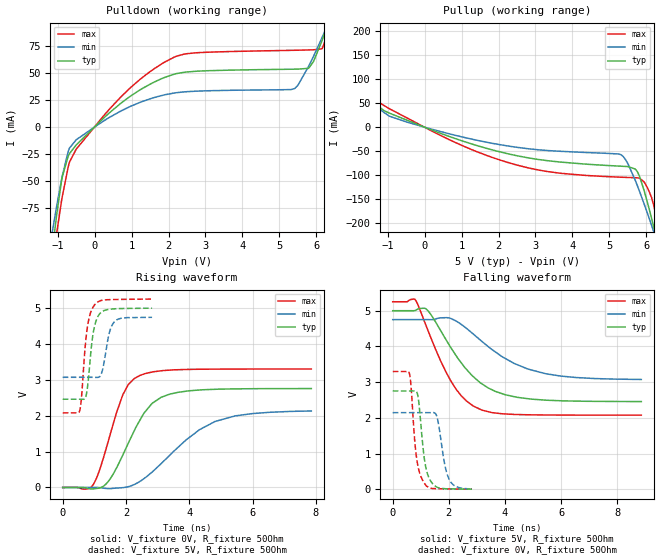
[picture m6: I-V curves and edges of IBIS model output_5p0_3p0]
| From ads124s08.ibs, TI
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|   output_5p0_3p0 Model
[Model]   output_5p0_3p0
Model_type   Output
Polarity   Non-Inverting
Vmeas = 2.5
Vref = 0
Cref = 2pF
Rref = 70
|   typ   min   max
|   (nom PVT)   (fast PVT)   (slow PVT)
C_comp   3.234e-12   3.122e-12   3.353e-12
| Where nom  PVT is Nominal Process, 5V, 27C
|   Fast PVT is Strong Process,  5.25V, -50C
|   Slow PVT is Weak Process,   4.75V, 125C
[Voltage Range]   5   4.75   5.25
|Junction Temperature
[Temperature Range]   27   125   -50
[Pullup Reference]   5   4.75   5.25
[Pulldown Reference]   0   0   0
[Power Clamp Reference]   5   4.75   5.25
[GND Clamp Reference]   0   0   0
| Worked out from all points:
|   slope of the pulldown table from 0 to 0.75 V, typ, clamps not added: 32.7 ohm
|   slope of the pullup table from 0 to 0.75 V, typ, clamps not added: 34.9 ohm
|   falling waveform, V_fixture 5V, R_fixture 50Ohm: 20-80 % time 1.48ns typ, 1.91ns min, 1.18ns max; typ from 5 V to 2.46 V
|   rising waveform, V_fixture 0V, R_fixture 50Ohm: 20-80 % time 988ps typ, 1.71ns min, 705ps max; typ from 0 V to 2.75 V
|   rising waveform, V_fixture 5V, R_fixture 50Ohm: 20-80 % time 199ps typ, 217ps min, 197ps max; typ from 2.46 V to 4.99 V
|   falling waveform, V_fixture 0V, R_fixture 50Ohm: 20-80 % time 237ps typ, 276ps min, 221ps max; typ from 2.75 V to 0.009 V
[Pulldown]
|   Voltage   I(typ)   I(min)   I(max)
-5V       -1.425A    -1.08A     -1.771A
-1.16V    -119.2mA   -100.1mA   -147mA
-1.015V   -78.19mA   -70.86mA   -95.57mA
-720mV    -27.41mA   -23.12mA   -37.56mA
-497mV    -16.44mA   -11.66mA   -20.31mA
905mV     27.09mA    18.18mA    34.43mA
2.225V    49.61mA    31.92mA    65.71mA
5.412V    53.62mA    35.7mA     71.12mA
5.79V     54.4mA     56.23mA    71.41mA
6.162V    80.92mA    83.39mA    72.89mA
6.403V    104.4mA    102.3mA    95.38mA
10V       508.4mA    415.8mA    608.3mA
[Pullup]
|   Voltage   I(typ)   I(min)   I(max)
-5V       423.9mA    339.6mA    534.5mA
-2.473V   163.8mA    135.3mA    202.2mA
-1.335V   51.05mA    46.44mA    59.22mA
-497mV    15.05mA    10.92mA    19.97mA
1.09V     -30.47mA   -21.72mA   -40.73mA
2.481V    -59.12mA   -41.74mA   -78.43mA
5.322V    -81.19mA   -57.63mA   -104mA
5.76V     -93.15mA   -122.3mA   -105.4mA
5.945V    -133.2mA   -160.7mA   -114.5mA
6.204V    -208.4mA   -218.2mA   -163.7mA
6.33V     -247.9mA   -247.6mA   -209.5mA
10V       -1.505A    -1.205A    -1.757A
[Ramp]
R_load = 50
|   typ   min   max
dV/dt_r   1.65274/9.88695e-10   1.28858/1.73231e-09   1.97906/7.04855e-10
dV/dt_f   1.52593/1.48214e-09   1.00955/1.93262e-09   1.90339/1.1769e-09
[Falling Waveform]
V_fixture = 5V
V_fixture_min = 4.75V
V_fixture_max = 5.25V
R_fixture = 50Ohm
|   Time   V(typ)   V(min)   V(max)
0s        5V         4.75V      5.25V
795.5ps   5.005V     4.75V      5.316V
1.22ns    5.027V     4.75V      4.519V
1.699ns   4.456V     4.8V       3.61V
2.076ns   3.959V     4.78V      3.027V
2.624ns   3.362V     4.508V     2.477V
3.173ns   2.956V     4.143V     2.219V
4.325ns   2.595V     3.525V     2.098V
5.445ns   2.497V     3.237V     2.082V
8.853ns   2.458V     3.076V     2.078V
[Rising Waveform]
V_fixture = 0V
V_fixture_min = 0V
V_fixture_max = 0V
R_fixture = 50Ohm
|   Time   V(typ)   V(min)   V(max)
0s        2.363nV    3.266nV    2.146nV
956.7ps   -39.32mV   138.3uV    71.13mV
1.416ns   142.2mV    -30.9mV    1.216V
1.897ns   898.8mV    -5.159mV   2.58V
2.076ns   1.241V     22.49mV    2.872V
2.447ns   1.886V     174.3mV    3.122V
3.112ns   2.512V     665.2mV    3.248V
3.898ns   2.68V      1.325V     3.285V
4.814ns   2.733V     1.838V     3.295V
7.853ns   2.753V     2.13V      3.298V
[Rising Waveform]
V_fixture = 5V
V_fixture_min = 4.75V
V_fixture_max = 5.25V
R_fixture = 50Ohm
|   Time   V(typ)   V(min)   V(max)
0s        2.457V     3.067V     2.078V
532.5ps   2.457V     3.067V     2.124V
589.1ps   2.456V     3.067V     2.466V
769.3ps   2.709V     3.068V     4.402V
927.3ps   4.081V     3.067V     4.969V
1.01ns    4.504V     3.066V     5.088V
1.22ns    4.881V     3.163V     5.206V
1.459ns   4.958V     4.26V      5.229V
1.635ns   4.974V     4.615V     5.233V
2.823ns   4.991V     4.737V     5.245V
[Falling Waveform]
V_fixture = 0V
V_fixture_min = 0V
V_fixture_max = 0V
R_fixture = 50Ohm
|   Time   V(typ)   V(min)   V(max)
0s        2.755V     2.148V     3.298V
589.1ps   2.755V     2.148V     3.26V
657.6ps   2.754V     2.148V     2.839V
795.5ps   2.757V     2.148V     1.255V
889.2ps   2.647V     2.148V     691.7mV
1.116ns   925.5mV    2.148V     183.5mV
1.302ns   302.7mV    2.147V     42.65mV
1.578ns   62.45mV    2.031V     19.33mV
2.014ns   16mV       268.2mV    13.04mV
2.823ns   8.804mV    15mV       6.958mV
